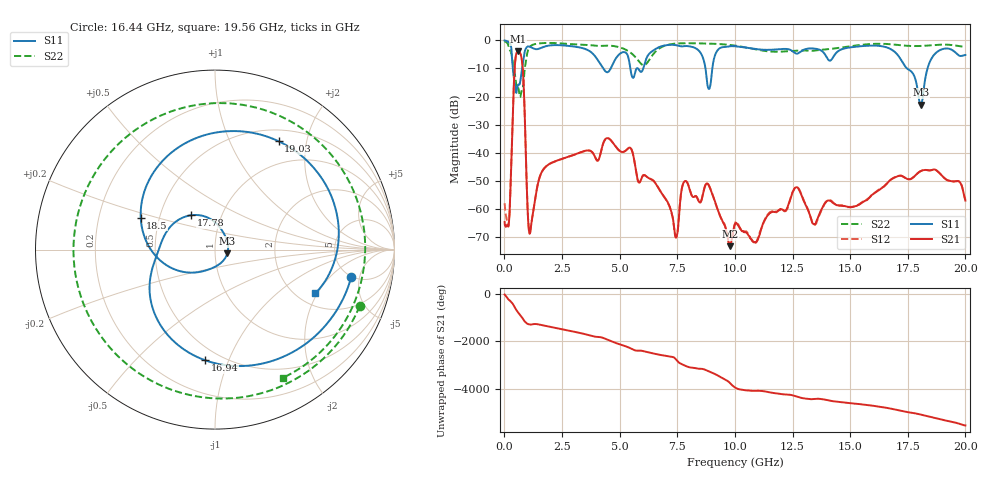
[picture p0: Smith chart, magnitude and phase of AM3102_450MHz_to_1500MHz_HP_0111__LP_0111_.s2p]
!Agilent Technologies,E8364B,MY43040894,A.07.50.67
!Agilent E8364B: A.07.50.67
!Date: Thursday, January 11, 2018 05:52:41
!Correction: S11(Full 2 Port(1,2))
!S21(Full 2 Port(1,2))
!S12(Full 2 Port(1,2))
!S22(Full 2 Port(1,2))
!S2P File: Measurements: S11, S21, S12, S22:
# Hz S  dB  R 50
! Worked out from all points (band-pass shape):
!   1601 points, 10 MHz to 20 GHz, reference 50 ohm
!   highest |S21| = -3.99 dB at 597.2 MHz (marker M1); lowest = -73.2 dB at 9.78 GHz (marker M2)
!   |S21| within 3 dB of the highest: 474.7 MHz to 757.4 MHz (282.7 MHz wide, 45.9 % of centre)
!   lowest |S11| = -22.9 dB at 18.06 GHz (marker M3), VSWR 1.15, Z = 57.3 - j2.5 ohm
!   |S11| at or under -10 dB: 365.4 MHz to 766.3 MHz (400.9 MHz wide, 70.9 % of centre); 4.288 GHz to 4.615 GHz (327.3 MHz wide, 7.35 % of centre); 17.46 GHz to 18.36 GHz (893.1 MHz wide, 4.99 % of centre)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
!   |S22| runs from -20.2 to -0.4 dB; largest |S21 - S12| = 0.0014
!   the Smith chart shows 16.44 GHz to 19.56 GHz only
!   S11 on the Smith chart (normalised r, x): 16.44 GHz: 4.90, -3.77; 16.94 GHz: 0.41, -0.83; 17.78 GHz: 0.71, +0.29; 18.5 GHz: 0.39, +0.18; 19.03 GHz: 0.65, +1.54; 19.56 GHz: 2.48, -1.92
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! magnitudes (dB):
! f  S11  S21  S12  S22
! 10 MHz  -0.1  -64.6  -58.0  -0.4
! 197.4 MHz  -0.7  -64.8  -64.5  -2.6
! 597.2 MHz  -15.8  -4.0  -4.0  -16.9
! 784.6 MHz  -9.0  -8.9  -8.9  -17.3
! 1.109 GHz  -2.3  -68.7  -68.3  -2.3
! 3.346 GHz  -2.7  -39.7  -39.7  -1.6
! 6.682 GHz  -2.5  -52.5  -52.5  -3.1
! 7.444 GHz  -1.7  -70.2  -70.1  -1.2
! 7.806 GHz  -2.1  -50.3  -50.2  -1.0
! 8.831 GHz  -16.7  -51.1  -51.0  -1.2
! 9.78 GHz  -2.1  -73.2  -72.7  -1.7
! 10.01 GHz  -2.1  -65.2  -65.0  -1.9
! 13.34 GHz  -2.9  -64.5  -64.4  -3.8
! 16.44 GHz  -2.2  -52.2  -52.2  -1.3
! 16.68 GHz  -2.8  -50.2  -50.3  -1.4
! 16.94 GHz  -4.2  -48.8  -48.7  -1.5
! 17.78 GHz  -12.6  -48.5  -48.4  -2.1
! 18.06 GHz  -22.9  -46.5  -46.5  -2.0
! 18.5 GHz  -6.9  -46.2  -46.2  -1.8
! 19.03 GHz  -3.1  -48.5  -48.5  -1.5
! 19.56 GHz  -4.3  -50.2  -50.1  -1.9
! 20 GHz  -5.2  -57.0  -56.7  -2.4
